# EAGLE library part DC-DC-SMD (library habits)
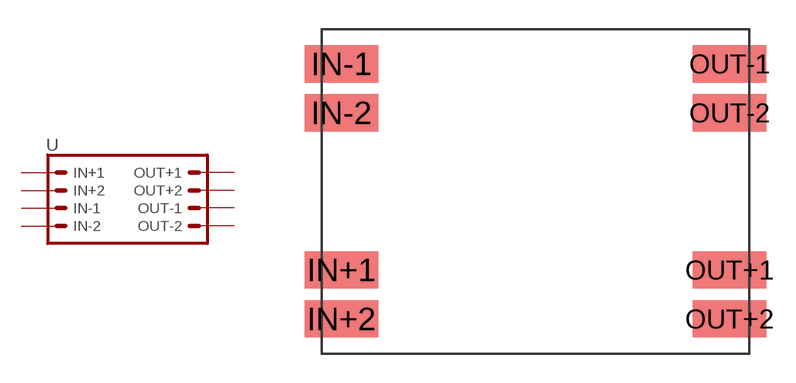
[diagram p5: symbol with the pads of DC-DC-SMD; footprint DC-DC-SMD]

Designator prefix -

## DC-DC-SMD  [DC-DC-SMD]
IN+1  IN+1  pas
IN+2  IN+2  pas
IN-1  IN-1  pas
IN-2  IN-2  pas
OUT+1  OUT+1  pas
OUT+2  OUT+2  pas
OUT-1  OUT-1  pas
OUT-2  OUT-2  pas

## Footprint DC-DC-SMD (pad centres in mm)
Plated Through Hole - 2x4 Specifications: Pin count:8 Pin pitch:0.1" Example device(s): CONN_04x2
smd 3.81 x 1.93: IN+1 -10.033,-4.065; IN+2 -10.033,-6.6; IN-1 -10.033,6.6; IN-2 -10.033,4.065; OUT+1 10.033,-4.065; OUT+2 10.033,-6.6; OUT-1 10.033,6.6; OUT-2 10.033,4.065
